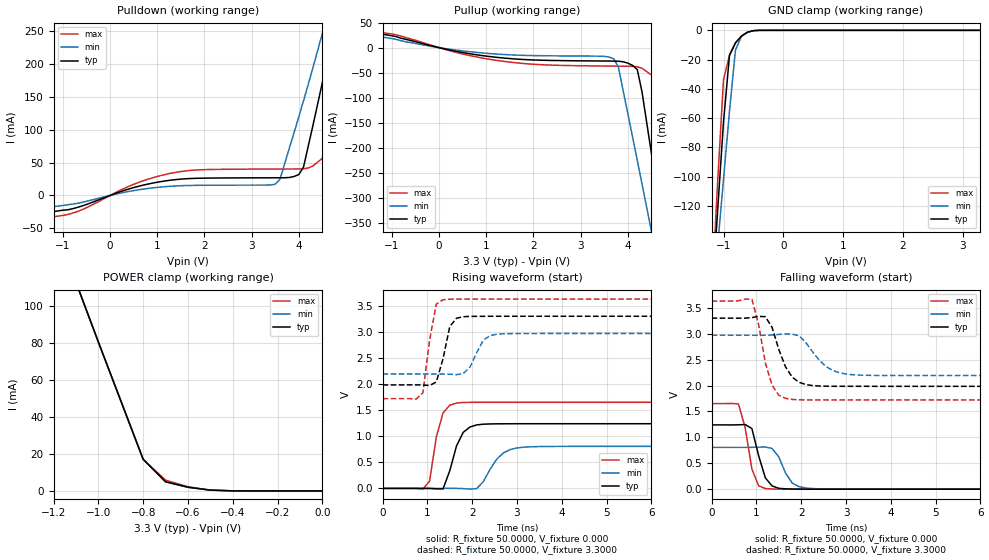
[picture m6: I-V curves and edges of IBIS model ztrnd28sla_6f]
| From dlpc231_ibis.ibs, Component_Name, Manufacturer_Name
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| Model ztrnd28sla_6f
[Model]   ztrnd28sla_6f
Model_type   I/O
Polarity   Non-Inverting
Enable   Active-High
Vinl = 0.8000V
Vinh = 2.0000V
Vmeas = 1.5000V
Cref =50.0000pF
Rref = 0.5000k
Vref =  0.000V
C_comp   0.7000pF   0.7000pF   0.7000pF
[Temperature Range]   25.0000   0.1240k   -40.0000
[Voltage Range]   3.3000V   2.9700V   3.6300V
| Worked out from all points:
|   slope of the pulldown table from 0 to 0.495 V, typ, clamps not added: 41.7 ohm
|   slope of the pullup table from 0 to 0.495 V, typ, clamps not added: 51.3 ohm
|   GND clamp passes 1 mA (typ) near -0.57 V on its own axis
|   POWER clamp passes 1 mA (typ) near -0.54 V on its own axis
|   rising waveform, R_fixture 50.0000, V_fixture 0.000: 20-80 % time 292ps typ, 385ps min, 226ps max; typ from 0 V to 1.24 V
|   rising waveform, R_fixture 50.0000, V_fixture 3.3000: 20-80 % time 215ps typ, 268ps min, 198ps max; typ from 1.98 V to 3.3 V
|   falling waveform, R_fixture 50.0000, V_fixture 0.000: 20-80 % time 238ps typ, 286ps min, 220ps max; typ from 1.24 V to 0 V
|   falling waveform, R_fixture 50.0000, V_fixture 3.3000: 20-80 % time 355ps typ, 476ps min, 288ps max; typ from 3.3 V to 1.98 V
[Pulldown]
-3.3V     -36mA      -27mA      -45mA
-900mV    -21.82mA   -14.1mA    -29.03mA
1.4V      24.15mA    14.48mA    35.22mA
3.5V      26.85mA    17.02mA    40.14mA
3.6V      26.87mA    24.59mA    40.16mA
4V        31.8mA     119.5mA    40.29mA
4.1V      43.22mA    144mA      40.49mA
4.5V      171.8mA    246.7mA    56.57mA
4.7V      239.3mA    301.4mA    133.3mA
4.9V      309.2mA    358.9mA    217.5mA
5.1V      382mA      420.2mA    304.4mA
6.6V      1.06A      974.8mA    1.071A
[Pullup]
-3.3V     22mA       27.8mA     15mA
-1.5V     31.7mA     25.8mA     34mA
1.2V      -19.14mA   -12.66mA   -25.2mA
3.7V      -26.85mA   -22.12mA   -36.91mA
3.8V      -27.1mA    -38.91mA   -36.99mA
4.2V      -43.73mA   -225.2mA   -38.15mA
4.3V      -88.01mA   -272.2mA   -41.21mA
4.5V      -211.3mA   -366.7mA   -54.54mA
4.7V      -335.7mA   -461.9mA   -116.1mA
4.9V      -460.9mA   -557.6mA   -272.3mA
5.1V      -586.9mA   -653.8mA   -429.5mA
6.6V      -1.543A    -1.386A    -1.621A
[GND_clamp]
-3.3V     -1.517A    -1.206A    -1.849A
-1.2V     -185.7mA   -194.8mA   -182.8mA
-1.1V     -124mA     -148.1mA   -104.8mA
-1V       -62.54mA   -101.7mA   -33.61mA
-900mV    -17.04mA   -55.16mA   -17.04mA
-800mV    -8.525mA   -13.45mA   -8.525mA
-700mV    -3.999mA   -3.999mA   -3.999mA
-600mV    -1.289mA   -1.289mA   -1.289mA
-500mV    -219.7uA   -252.6uA   -203.6uA
-400mV    -15.61uA   -27.49uA   -11.15uA
3.3V      3.373nA    3.373nA    17.05nA
[POWER_clamp]
-3.3V     1.027A     840.1mA    1.22A
-1.1V     112.7mA    112.7mA    112.7mA
-1V       80.41mA    80.41mA    80.41mA
-800mV    17.08mA    17.08mA    17.08mA
-700mV    4.947mA    4.947mA    5.794mA
-600mV    1.98mA     1.98mA     2.27mA
-500mV    443.8uA    443.8uA    443.8uA
-400mV    34.78uA    34.78uA    34.78uA
0V        3.373nA    3.373nA    57.43nA
[Ramp]
dV/dt_r   0.7440/0.2666n   0.4834/0.3752n   0.9906/0.2060n
dV/dt_f   0.7896/0.3427n   0.4662/0.4703n   1.1454/0.2689n
R_load = 50.0000
[Rising Waveform]
R_fixture = 50.0000
V_fixture = 0.000
V_fixture_min = 0.000
V_fixture_max = 0.000
0s        0V         0V         0V
900ps     205.4uV    -1.838uV   -14.61mV
1.05ns    361.8uV    -4.159uV   140.1mV
1.2ns     -8.739mV   -3.876uV   985.1mV
1.35ns    -8.955mV   66.32uV    1.446V
1.65ns    812.7mV    293.6uV    1.636V
1.95ns    1.177V     -12.53mV   1.65V
2.7ns     1.239V     681.4mV    1.651V
3.15ns    1.24V      790.3mV    1.651V
14.85ns   1.24V      805.7mV    1.651V
[Rising Waveform]
R_fixture = 50.0000
V_fixture = 3.3000
V_fixture_min = 2.9700
V_fixture_max = 3.6300
0s        1.984V     2.193V     1.721V
900ps     1.983V     2.193V     1.832V
1.05ns    1.972V     2.193V     2.845V
1.2ns     2.041V     2.193V     3.534V
1.35ns    2.487V     2.192V     3.617V
1.5ns     3.103V     2.189V     3.628V
1.8ns     3.292V     2.201V     3.629V
2.25ns    3.299V     2.844V     3.63V
2.7ns     3.3V       2.964V     3.63V
14.85ns   3.3V       2.97V      3.63V
[Falling Waveform]
R_fixture = 50.0000
V_fixture = 0.000
V_fixture_min = 0.000
V_fixture_max = 0.000
0s        1.24V      805.7mV    1.651V
600ps     1.242V     805.6mV    1.644V
750ps     1.247V     805.5mV    1.186V
900ps     1.169V     806.7mV    386.1mV
1.05ns    647.4mV    810.5mV    64.82mV
1.2ns     217.5mV    814.1mV    11.85mV
1.5ns     16.52mV    622.9mV    1.158mV
1.8ns     2.707mV    117mV      102.6uV
2.25ns    164uV      11.41mV    2.481uV
14.85ns   0V         0V         0V
[Falling Waveform]
R_fixture = 50.0000
V_fixture = 3.3000
V_fixture_min = 2.9700
V_fixture_max = 3.6300
0s        3.3V       2.97V      3.63V
900ps     3.311V     2.969V     3.664V
1.05ns    3.334V     2.969V     3.177V
1.2ns     3.328V     2.97V      2.439V
1.35ns    3.122V     2.973V     2.004V
1.65ns    2.36V      2.995V     1.751V
1.8ns     2.161V     2.991V     1.731V
2.55ns    1.987V     2.37V      1.721V
3.15ns    1.985V     2.208V     1.721V
14.85ns   1.984V     2.193V     1.721V
